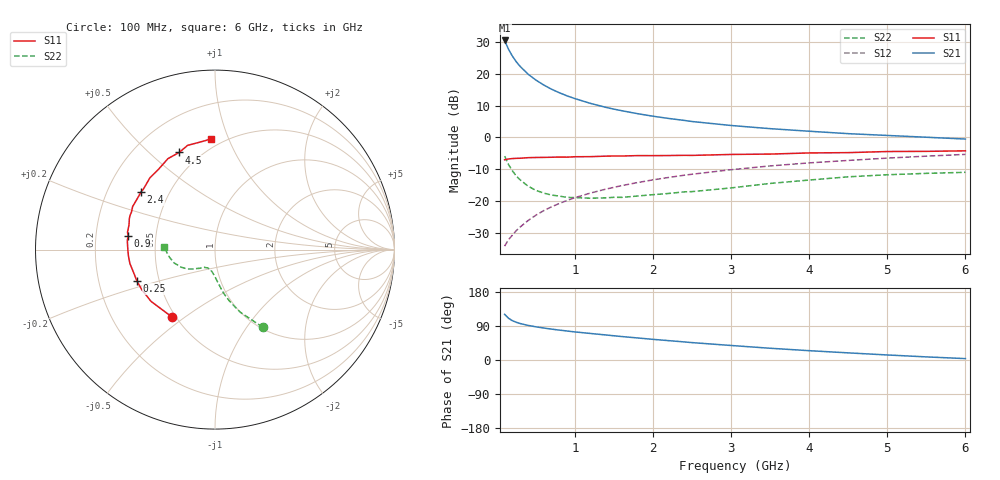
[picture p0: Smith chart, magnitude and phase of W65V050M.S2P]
! SIEMENS Small Signal Semiconductors
! BFR193W
! Si NPN RF Bipolar Junction Transistor in SOT323
! VCE = 5 V  IC = 50 mA
! Common Emitter S-Parameters:  September  1992
# GHz  S  MA  R  50
!  f  S11  S21  S12  S22
! GHz  MAG  ANG  MAG  ANG  MAG  ANG  MAG  ANG
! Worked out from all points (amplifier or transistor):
!   28 points, 100 MHz to 6 GHz, reference 50 ohm
!   highest |S21| = 30.6 dB at 100 MHz (marker M1)
!   |S21| within 3 dB of that: start of sweep to 155.2 MHz
!   unconditionally stable (mu >= 1): 538.4 MHz to 2.592 GHz
!   at 300 MHz: K = 0.92, MSG = 25.3 dB, |S12| = -28.2 dB
!   at 1.5 GHz: K = 1.03, MAG = 11.3 dB, |S12| = -15.7 dB
!   at 6 GHz: K = 0.92, MSG = 2.4 dB, |S12| = -5.3 dB
!   S11 on the Smith chart (normalised r, x): 100 MHz: 0.48, -0.45; 250 MHz: 0.37, -0.17; 900 MHz: 0.34, +0.07; 2.4 GHz: 0.35, +0.31; 4.5 GHz: 0.39, +0.63; 6 GHz: 0.43, +0.86
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0.1  0.4454 -122.7  33.93 120.6  0.0193 60.9  0.5078 -58.4
0.15  0.4586 -141.1  24.66 110.2  0.0245 62.0  0.3743 -68.2
0.2  0.4651 -151.4  19.18 103.7  0.0288 64.4  0.298 -74.3
0.25  0.469 -158.2  15.62 99.5  0.034 66.0  0.2462 -79.0
0.3  0.4704 -163.3  13.18 96.2  0.0388 67.8  0.2143 -81.7
0.4  0.4804 -170.7  9.988 91.3  0.0489 70.4  0.1708 -86.8
0.5  0.4836 -175.7  8.051 87.6  0.0594 71.5  0.1467 -90.7
0.6  0.4853 -179.7  6.743 84.4  0.0701 72.2  0.1328 -95.0
0.7  0.4878 177.1  5.78 81.5  0.0805 72.6  0.1236 -97.7
0.8  0.4912 174.0  5.086 78.9  0.091 72.5  0.119 -101.0
0.9  0.4895 171.3  4.531 76.5  0.1017 72.2  0.1136 -103.2
1  0.4969 168.8  4.107 74.1  0.1123 71.9  0.1125 -105.6
1.2  0.4985 163.9  3.449 70.0  0.133 71.0  0.1102 -111.6
1.4  0.5078 160.0  2.981 66.0  0.1536 69.9  0.1116 -115.5
1.6  0.5102 155.7  2.644 61.9  0.1741 68.5  0.1136 -119.7
2.2  0.5191 144.9  1.997 51.1  0.2341 64.0  0.1309 -128.1
2.4  0.5231 142.0  1.859 47.7  0.254 62.4  0.1388 -130.8
3  0.5401 132.1  1.546 38.3  0.3102 57.3  0.1602 -137.6
3.5  0.5473 125.0  1.378 31.0  0.356 52.8  0.1885 -145.1
4.5  0.577 110.2  1.149 18.8  0.4346 44.2  0.2397 -162.0
5.5  0.6042 98.3  1.009 8.2  0.5076 35.8  0.2718 -178.1
6  0.616 92.3  0.945 3.7  0.5412 31.5  0.2821 177.4
